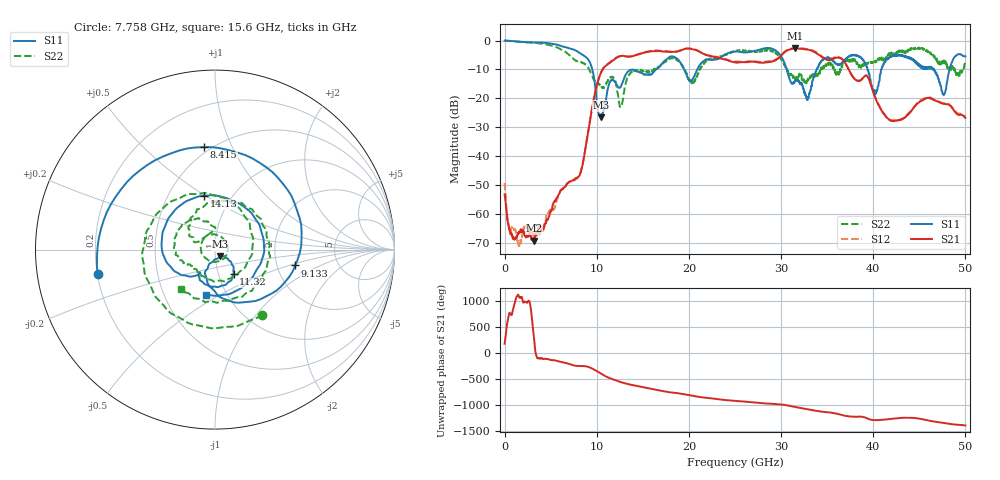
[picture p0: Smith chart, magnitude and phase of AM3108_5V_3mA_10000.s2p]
# Hz S DB R 50.0
!freq dBS11 angS11 dBS21 angS21 dBS12 angS12 dBS22 angS22
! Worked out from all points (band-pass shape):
!   1601 points, 10 MHz to 50 GHz, reference 50 ohm
!   highest |S21| = -2.72 dB at 31.53 GHz (marker M1); lowest = -69.3 dB at 3.197 GHz (marker M2)
!   |S21| within 3 dB of the highest: 12.28 GHz to 22.85 GHz (10.57 GHz wide, 60.2 % of centre); 29.86 GHz to 34.45 GHz (4.584 GHz wide, 14.3 % of centre)
!   lowest |S11| = -26.5 dB at 10.48 GHz (marker M3), VSWR 1.10, Z = 52.9 - j3.9 ohm
!   |S11| at or under -10 dB: 9.527 GHz to 16.45 GHz (6.924 GHz wide, 53.3 % of centre); 30.62 GHz to 33.85 GHz (3.228 GHz wide, 10 % of centre); 46.62 GHz to 48.29 GHz (1.671 GHz wide, 3.52 % of centre)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
!   |S22| runs from -23.2 to 0.0 dB; largest |S21 - S12| = 0.027
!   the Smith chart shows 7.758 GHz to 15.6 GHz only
!   S11 on the Smith chart (normalised r, x): 7.758 GHz: 0.20, -0.10; 8.415 GHz: 0.46, +0.79; 9.133 GHz: 2.53, -0.57; 11.32 GHz: 1.18, -0.33; 14.13 GHz: 0.75, +0.49; 15.6 GHz: 0.80, -0.43
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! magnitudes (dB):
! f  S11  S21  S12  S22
! 10 MHz  0.0  -53.3  -49.3  0.0
! 1.541 GHz  -0.4  -66.3  -71.2  -0.4
! 3.197 GHz  -0.7  -69.3  -67.8  -0.7
! 7.758 GHz  -3.5  -47.6  -48.0  -6.9
! 8.352 GHz  -4.7  -44.7  -44.3  -7.5
! 8.415 GHz  -4.8  -43.8  -43.5  -7.7
! 9.133 GHz  -6.8  -30.4  -30.3  -9.8
! 10.48 GHz  -26.5  -11.0  -11.0  -15.6
! 11.32 GHz  -15.3  -7.9  -7.8  -13.1
! 12.63 GHz  -15.8  -5.3  -5.3  -22.9
! 14.13 GHz  -10.3  -5.2  -5.1  -10.2
! 15.6 GHz  -11.7  -3.9  -3.8  -10.8
! 16.69 GHz  -9.4  -3.6  -3.5  -9.4
! 20.41 GHz  -13.3  -3.0  -2.9  -14.8
! 25 GHz  -3.8  -7.6  -7.3  -3.7
! 31.53 GHz  -14.1  -2.7  -2.6  -13.7
! 33.35 GHz  -15.5  -3.5  -3.3  -12.7
! 38 GHz  -4.9  -13.4  -13.3  -6.6
! 40.22 GHz  -18.6  -19.9  -19.6  -7.6
! 41.69 GHz  -6.0  -27.3  -27.1  -5.2
! 47.66 GHz  -18.9  -21.9  -21.7  -7.7
! 50 GHz  -5.5  -26.7  -26.4  -6.9
